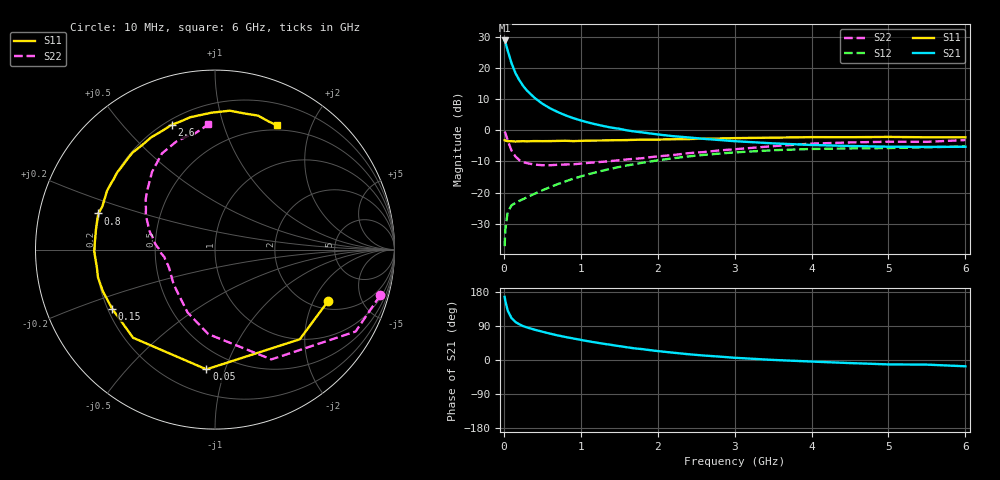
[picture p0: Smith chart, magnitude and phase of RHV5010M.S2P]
! SIEMENS Small Signal Semiconductors
! BFR106
! Si NPN RF Bipolar Junction Transistor in SOT23
! VCE = 0.5 V  IC = 10 mA
! Common Emitter S-Parameters:  August  1996
# GHz  S  MA  R  50
!  f  S11  S21  S12  S22
! GHz  MAG  ANG  MAG  ANG  MAG  ANG  MAG  ANG
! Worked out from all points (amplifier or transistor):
!   36 points, 10 MHz to 6 GHz, reference 50 ohm
!   highest |S21| = 28.9 dB at 10 MHz (marker M1)
!   |S21| within 3 dB of that: start of sweep to 47.21 MHz
!   unconditionally stable (mu >= 1): 433.9 MHz to end of sweep
!   at 250 MHz: K = 0.75, MSG = 18.2 dB, |S12| = -22.1 dB
!   at 1.4 GHz: K = 1.14, MAG = 4.3 dB, |S12| = -12.3 dB
!   at 6 GHz: K = 1.03, MAG = -1.1 dB, |S12| = -5.2 dB
!   S11 on the Smith chart (normalised r, x): 10 MHz: 2.39, -2.63; 50 MHz: 0.36, -0.86; 150 MHz: 0.22, -0.25; 800 MHz: 0.19, +0.15; 2.6 GHz: 0.23, +0.69; 6 GHz: 0.44, +1.53
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0.01  0.693 -24.3  27.77 166.7  0.0138 79.8  0.9551 -15.5
0.02  0.6876 -46.6  26.12 155.5  0.0257 69.4  0.9068 -30.2
0.05  0.6689 -94.1  19.1 130.5  0.0487 49.3  0.6878 -62.8
0.1  0.6705 -132.9  11.97 110.7  0.0626 38.0  0.4725 -94.5
0.15  0.661 -150.2  8.372 100.5  0.0684 35.7  0.3824 -113.5
0.2  0.6667 -159.7  6.446 94.4  0.0736 36.8  0.3332 -125.1
0.25  0.6702 -166.6  5.187 89.5  0.0785 38.9  0.3085 -135.2
0.3  0.6656 -171.3  4.36 86.0  0.0839 41.2  0.2974 -141.5
0.4  0.6731 -179.1  3.322 80.0  0.096 44.9  0.2818 -151.1
0.5  0.6706 175.8  2.683 74.7  0.1086 47.7  0.2757 -157.6
0.6  0.6726 170.7  2.265 69.6  0.1227 49.7  0.2755 -161.9
0.7  0.676 166.3  1.97 64.9  0.1369 51.2  0.2798 -165.5
0.8  0.6806 162.8  1.745 60.8  0.1514 51.8  0.2828 -168.9
1.1  0.685 151.4  1.333 49.3  0.1973 51.7  0.3007 -176.1
1.3  0.6879 144.9  1.17 42.7  0.2276 50.2  0.3135 179.0
1.6  0.6982 136.1  0.999 33.6  0.273 47.0  0.3408 172.7
2.2  0.7195 119.7  0.806 19.3  0.3561 38.5  0.4012 158.9
2.6  0.736 109.2  0.73 11.8  0.4034 32.0  0.4481 149.2
3.5  0.763 91.5  0.618 0.2  0.4795 17.6  0.5574 129.0
4.5  0.776 77.6  0.561 -8.1  0.5122 3.4  0.6394 109.7
5.5  0.7738 67.3  0.542 -12.2  0.5356 -4.9  0.6539 100.3
6  0.7738 63.4  0.545 -16.6  0.5503 -11.1  0.6983 93.0
